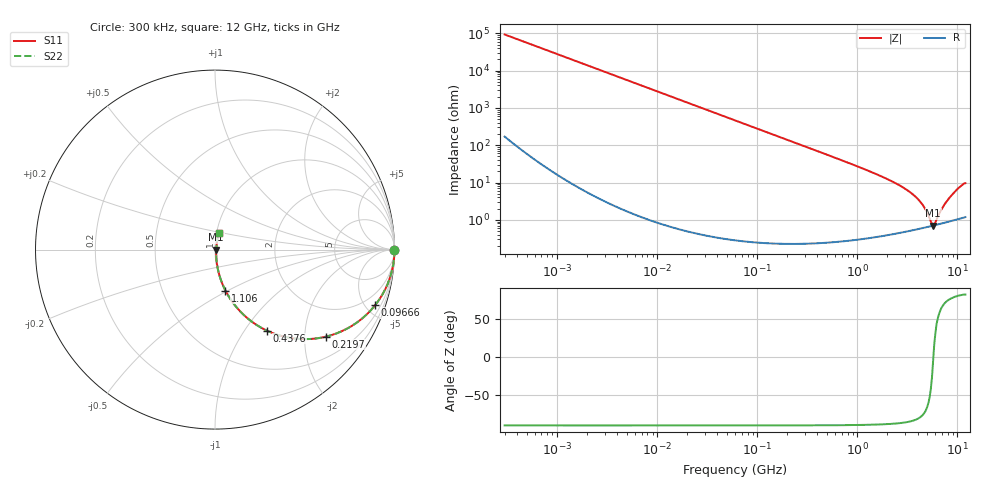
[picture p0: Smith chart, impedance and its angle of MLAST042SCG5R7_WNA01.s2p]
! MLAST042SCG5R7_WNA01  S-PARAMETER MODEL  ( General Type )
! Model Generated by TAIYO YUDEN Corporation (http://www.ty-top.com)
! Version 1.0
! TAIYO YUDEN Control No. 150820
! Copyright(c) 2015 TAIYO YUDEN CO.,LTD. All Rights Reserved.
! Product Description (link to TY-COMPAS)
! https://ds.yuden.co.jp/TYCOMPAS/or/detail?pn=MLAST042SCG5R7BWNA01&u=M
! Products Name : Multilayer Ceramic Capacitors
! Characteristics :
!  Capacitance : 5.7 pF , Rated Voltage : 25V , TCC : CG / C0G
!  Case Size : 0.4 x 0.2 / 0.016 x 0.008 [mm/inch] , Thickness : 0.2 / 0.008 [mm/inch]
!  (Conditions: Temperature = 25 degC , DC Bias Current/Voltage = 0A / 0V)
! External Node Assignments :
!  1  o---| |---o  2
! GND o---------o GND
! Frequency Range : 0.3MHz  -  12000MHz  [ 401 STEP ]
# MHz S RI R 50
! Freq[MHz].  S11 Real  S11 Imag  S21 Real  S21 Imag  S12 Real  S12 Imag  S22 Real  S22 Imag
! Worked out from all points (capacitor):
!   401 points, 300 kHz to 12 GHz, reference 50 ohm
!   read as one part in series: C = 5.69 pF near 316.3 kHz
!   lowest |Z| = 701 mohm at 5.715 GHz (marker M1)
!   series resonance near 5.747 GHz, so ESL is about 130 pH
!   S11 on the Smith chart (normalised r, x): 300 kHz: open; 96.66 MHz: 1.00, -5.78; 219.7 MHz: 1.00, -2.54; 437.6 MHz: 1.00, -1.27; 1.106 GHz: 1.01, -0.49; 12 GHz: 1.02, +0.19
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0.3  1 -0.00107  3.11e-06 0.00107  3.11e-06 0.00107  1 -0.00107
1.769972  1 -0.00633  4.27e-05 0.00633  4.27e-05 0.00633  1 -0.00633
10.44266  0.9986 -0.0373  0.00141 0.0373  0.00141 0.0373  0.9986 -0.0373
27.82928  0.9901 -0.0986  0.00985 0.0986  0.00985 0.0986  0.9901 -0.0986
60  0.9558 -0.2052  0.0442 0.2052  0.0442 0.2052  0.9558 -0.2052
96.65937  0.8929 -0.3088  0.1071 0.3088  0.1071 0.3088  0.8929 -0.3088
219.7372  0.6172 -0.4852  0.3828 0.4852  0.3828 0.4852  0.6172 -0.4852
353.9943  0.3826 -0.4846  0.6174 0.4846  0.6174 0.4846  0.3826 -0.4846
437.5599  0.2882 -0.451  0.7118 0.451  0.7118 0.451  0.2882 -0.451
686.4755  0.1404 -0.3442  0.8596 0.3442  0.8596 0.3442  0.1404 -0.3442
1105.905  0.0585 -0.2285  0.9415 0.2285  0.9415 0.2285  0.0585 -0.2285
2088.533  0.0171 -0.1138  0.9829 0.1138  0.9829 0.1138  0.0171 -0.1138
3026.31  0.00914 -0.066  0.9909 0.066  0.9909 0.066  0.00914 -0.066
3944.255  0.00691 -0.0372  0.9931 0.0372  0.9931 0.0372  0.00691 -0.0372
4623.766  0.00652 -0.0213  0.9935 0.0213  0.9935 0.0213  0.00652 -0.0213
5420.343  0.00674 -0.0059  0.9933 0.0059  0.9933 0.0059  0.00674 -0.0059
5715.274  0.00694 -0.000596  0.9931 0.000596  0.9931 0.000596  0.00694 -0.000596
6026.253  0.0072 0.00452  0.9928 -0.00452  0.9928 -0.00452  0.0072 0.00452
7064.448  0.00834 0.0189  0.9917 -0.0189  0.9917 -0.0189  0.00834 0.0189
8281.503  0.0103 0.0367  0.9897 -0.0367  0.9897 -0.0367  0.0103 0.0367
10236.47  0.0151 0.0683  0.9849 -0.0683  0.9849 -0.0683  0.0151 0.0683
12000  0.0203 0.0922  0.9797 -0.0922  0.9797 -0.0922  0.0203 0.0922
